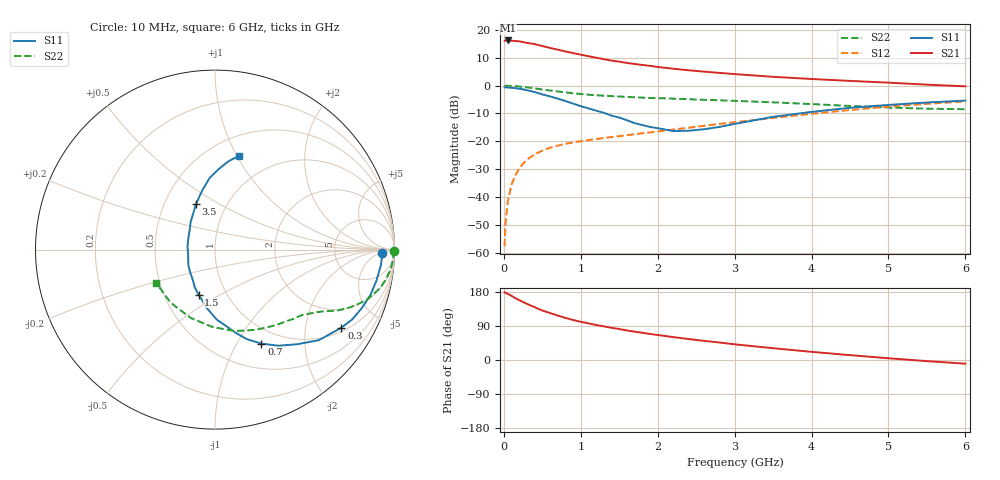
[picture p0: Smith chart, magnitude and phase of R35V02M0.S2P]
! SIEMENS Small Signal Semiconductors
! BFR181
! Si NPN RF Bipolar Junction Transistor in SOT23
! VCE = 5 V  IC = 2 mA
! Common Emitter S-Parameters:  May  1996
# GHz  S  MA  R  50
!  f  S11  S21  S12  S22
! GHz  MAG  ANG  MAG  ANG  MAG  ANG  MAG  ANG
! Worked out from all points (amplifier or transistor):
!   36 points, 10 MHz to 6 GHz, reference 50 ohm
!   highest |S21| = 16.3 dB at 50 MHz (marker M1)
!   |S21| within 3 dB of that: start of sweep to 651.7 MHz
!   unconditionally stable (mu >= 1): 1.626 GHz to 3.384 GHz
!   at 250 MHz: K = 0.23, MSG = 21.8 dB, |S12| = -28.0 dB
!   at 1.4 GHz: K = 0.94, MSG = 13.7 dB, |S12| = -18.5 dB
!   at 6 GHz: K = 0.86, MSG = 2.7 dB, |S12| = -5.7 dB
!   lowest NFmin = 1.35 dB at 450 MHz
!   S11 on the Smith chart (normalised r, x): 10 MHz: 25, -7; 300 MHz: 1.14, -3.14; 700 MHz: 0.80, -1.27; 1.5 GHz: 0.74, -0.40; 3.5 GHz: 0.72, +0.39; 6 GHz: 0.69, +1.02
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0.01  0.9299 -1.2  6.448 178.9  0.0013 86.3  0.9968 -0.5
0.02  0.9329 -2.0  6.393 177.5  0.0031 87.3  0.9919 -1.1
0.05  0.9278 -5.6  6.497 174.5  0.0081 87.6  0.9945 -2.6
0.1  0.9156 -11.0  6.426 169.3  0.0167 83.5  0.9879 -5.2
0.15  0.9018 -16.4  6.339 163.1  0.0246 80.0  0.9778 -7.7
0.2  0.8806 -21.7  6.272 158.0  0.0321 77.3  0.9642 -10.2
0.3  0.8275 -31.7  5.879 148.1  0.0467 71.7  0.9319 -14.3
0.4  0.7678 -41.1  5.591 139.4  0.058 66.7  0.8942 -18.0
0.5  0.6971 -49.2  5.152 130.6  0.0678 63.3  0.8523 -20.9
0.7  0.5844 -63.7  4.446 117.3  0.0832 58.2  0.7853 -25.1
0.8  0.5298 -70.4  4.121 111.2  0.0902 56.2  0.757 -26.7
0.9  0.4766 -76.2  3.855 105.6  0.0955 55.1  0.7302 -27.9
1.1  0.3906 -88.5  3.389 96.7  0.1049 54.1  0.688 -30.1
1.3  0.3252 -98.8  2.989 88.8  0.1146 53.5  0.6595 -32.0
1.5  0.2669 -110.1  2.699 81.8  0.1237 53.6  0.6378 -33.9
1.8  0.1957 -132.7  2.355 71.8  0.1391 54.7  0.6097 -36.6
2.2  0.1528 -167.8  2.018 60.5  0.162 55.5  0.5837 -41.3
3  0.2052 131.3  1.615 41.4  0.2194 55.3  0.5332 -52.9
3.5  0.2753 112.6  1.442 31.1  0.2631 53.3  0.501 -63.2
4.5  0.4002 94.3  1.218 12.8  0.3656 45.3  0.4311 -92.0
5.5  0.4981 81.3  1.042 -3.0  0.4716 33.1  0.3855 -129.6
6  0.539 75.7  0.973 -9.7  0.5208 25.8  0.377 -150.0
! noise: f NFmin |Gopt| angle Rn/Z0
0.45  1.35  0.6  17  0.4
0.9  1.45  0.5  36  0.4
1.8  1.8  0.31  80  0.37
